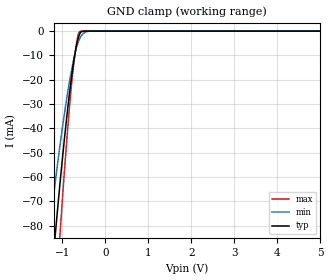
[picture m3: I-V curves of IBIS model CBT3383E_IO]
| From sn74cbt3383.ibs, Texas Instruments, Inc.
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[Model]   CBT3383E_IO
Model_type  Terminator
| variable   typ   min   max
C_comp   5.03pF   4.12pF   8.19pF
| C_tri-state   5.03pF   4.12pF   8.19pF
[Temperature Range]   40   100   -40
| Ambient temperature   25   85   -40
[Voltage range]   5   4.5   5.5
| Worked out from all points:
|   GND clamp passes 1 mA (typ) near -0.59 V on its own axis
[GND Clamp]
| CBT3383E_IO
|   Voltage   I(typ)   I(min)   I(max)
-5V       -1.102A    -854.2mA   -1.435A
-1.305V   -112mA     -82.53mA   -152.3mA
-1.17V    -84.38mA   -62.56mA   -114mA
-1.13V    -76.54mA   -56.93mA   -103.1mA
-1.05V    -61.41mA   -46.11mA   -81.83mA
-895mV    -34.66mA   -27.21mA   -43.96mA
-785mV    -18.51mA   -15.82mA   -21.46mA
-670mV    -5.714mA   -6.608mA   -4.763mA
-595mV    -1.075mA   -2.93mA    -111.6uA
-480mV    -29.73uA   -550.1uA   -823.4nA
-330mV    -245.9nA   -17.3uA    -2.419nA
5V        91.28pA    2.248nA    51.41pA
